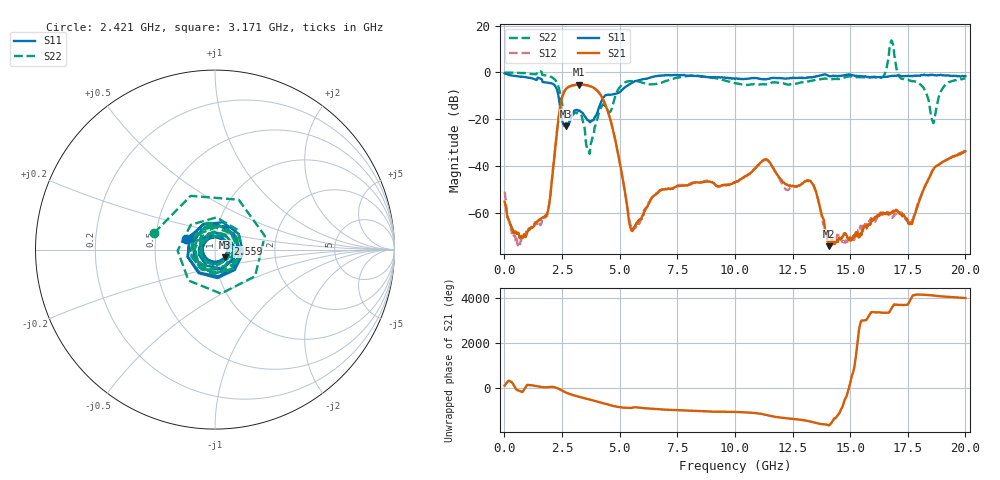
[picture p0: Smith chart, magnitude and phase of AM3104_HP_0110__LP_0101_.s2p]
!Created with skrf (http://scikit-rf.org).
# Hz S RI R 50.0
!freq ReS11 ImS11 ReS21 ImS21 ReS12 ImS12 ReS22 ImS22
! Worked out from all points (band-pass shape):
!   1601 points, 10 MHz to 20 GHz, reference 50 ohm
!   highest |S21| = -5.16 dB at 3.246 GHz (marker M1); lowest = -74.0 dB at 14.08 GHz (marker M2)
!   |S21| within 3 dB of the highest: 2.596 GHz to 4.07 GHz (1.473 GHz wide, 44.2 % of centre)
!   lowest |S11| = -22.9 dB at 2.684 GHz (marker M3), VSWR 1.15, Z = 55.7 - j4.91 ohm
!   |S11| at or under -10 dB: 2.347 GHz to 4.352 GHz (2.005 GHz wide, 59.9 % of centre)
!   |S22| runs from -34.7 to 13.6 dB; largest |S21 - S12| = 0.03
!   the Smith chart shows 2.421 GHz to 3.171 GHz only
!   S11 on the Smith chart (normalised r, x): 2.421 GHz: 0.72, +0.08; 2.559 GHz: 1.15, +0.07; 3.171 GHz: 0.75, +0.10
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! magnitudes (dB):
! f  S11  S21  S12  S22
! 10 MHz  -0.4  -55.0  -50.7  0.0
! 584.7 MHz  -1.6  -68.6  -73.6  -0.1
! 1.797 GHz  -4.2  -61.2  -61.2  -1.2
! 2.421 GHz  -15.4  -14.6  -14.6  -9.1
! 2.559 GHz  -22.0  -9.0  -9.0  -16.2
! 2.684 GHz  -22.9  -6.9  -6.9  -21.3
! 3.171 GHz  -16.1  -5.2  -5.3  -17.1
! 3.246 GHz  -16.4  -5.2  -5.2  -17.5
! 3.346 GHz  -16.9  -5.2  -5.3  -18.3
! 3.658 GHz  -20.5  -5.7  -5.8  -33.1
! 4.458 GHz  -9.5  -15.6  -15.6  -15.6
! 5.52 GHz  -4.4  -67.3  -66.8  -3.7
! 6.682 GHz  -1.4  -50.9  -50.7  -4.7
! 10.01 GHz  -2.7  -46.9  -46.7  -4.6
! 11.33 GHz  -2.9  -37.0  -37.3  -5.1
! 13.34 GHz  -2.1  -47.1  -47.1  -3.5
! 14.08 GHz  -1.5  -74.0  -68.9  -2.9
! 16.35 GHz  -1.9  -60.2  -59.7  -2.3
! 16.68 GHz  -1.6  -59.9  -60.6  7.2
! 17.64 GHz  -1.5  -64.0  -63.6  -3.6
! 18.59 GHz  -1.0  -41.6  -41.8  -21.2
! 20 GHz  -1.5  -33.6  -33.2  -2.5
